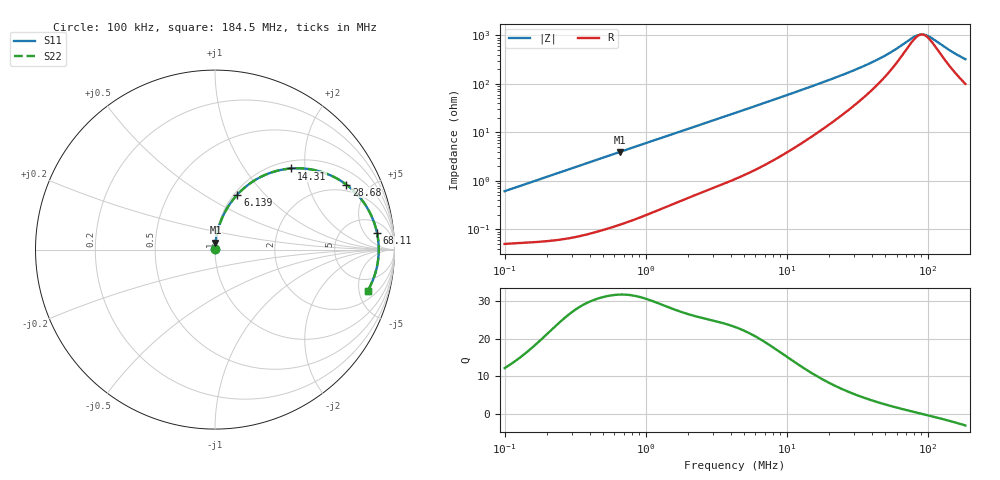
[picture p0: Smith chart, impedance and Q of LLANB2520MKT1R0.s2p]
! LLANB2520MKT1R0  S-PARAMETER MODEL  ( General Type )
! Model Generated by TAIYO YUDEN Corporation (http://www.ty-top.com)
! Version 2.0
! TAIYO YUDEN Control No. 20210629
! Copyright(c) 2012 TAIYO YUDEN CO.,LTD. All Rights Reserved.
! Product Description (link to TY-COMPAS)
! https://ds.yuden.co.jp/TYCOMPAS/or/detail?pn=LLANB2520MKT1R0M&u=M
! Products Name : Inductors
! Characteristics :
!  Inductance : 1.0 uH , SRF(min) : -Hz , DC Resistance(max) : 0.059 Ohm
!  Rated Current : Saturation :3100 mA , Temp Rise : 2700 mA (40 degC)
!  Case Size : 2.5 x 2.0 / 0.098 x 0.079 [mm/inch] , Thickness : 1.2 / 0.047 [mm/inch]
!  (Conditions: Temperature = 25 degC , DC Bias Current/Voltage = 0A / 0V)
! External Node Assignments :
!  1  o---GGG---o  2
! GND o---------o GND
! Frequency Range : 0.1MHz  -  184.468258MHz  [ 402 STEP ]
# MHz S RI R 50
! Freq[MHz].  S11 Real  S11 Imag  S21 Real  S21 Imag  S12 Real  S12 Imag  S22 Real  S22 Imag
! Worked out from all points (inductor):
!   401 points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, 100 kHz to 184.5 MHz, reference 50 ohm
!   read as one part in series: L = 966 nH near 103.8 kHz
!   highest Q = 31.7 at 655.4 kHz (marker M1), where L = 956 nH
!   self-resonance near 90.66 MHz
!   S11 on the Smith chart (normalised r, x): 100 kHz: 1.00, +0.01; 6.139 MHz: 1.03, +0.71; 14.31 MHz: 1.15, +1.68; 28.68 MHz: 1.64, +3.56; 68.11 MHz: 10, +10; 184.5 MHz: 2.99, -6.13
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0.1  0.000536 0.00607  0.9995 -0.00607  0.9995 -0.00607  0.000536 0.00607
0.352405  0.00119 0.0212  0.9988 -0.0212  0.9988 -0.0212  0.00119 0.0212
0.655361  0.00278 0.0392  0.9972 -0.0392  0.9972 -0.0392  0.00278 0.0392
1.241892  0.00791 0.0732  0.9921 -0.0732  0.9921 -0.0732  0.00791 0.0732
2.398015  0.0246 0.1367  0.9754 -0.1367  0.9754 -0.1367  0.0246 0.1367
4.294977  0.0678 0.2307  0.9322 -0.2307  0.9322 -0.2307  0.0678 0.2307
6.138922  0.1248 0.3069  0.8752 -0.3069  0.8752 -0.3069  0.1248 0.3069
9.283629  0.2403 0.3973  0.7597 -0.3973  0.7597 -0.3973  0.2403 0.3973
14.30567  0.4228 0.4519  0.5772 -0.4519  0.5772 -0.4519  0.4228 0.4519
15.13571  0.4497 0.4532  0.5503 -0.4532  0.5503 -0.4532  0.4497 0.4532
20.44747  0.5926 0.4332  0.4074 -0.4332  0.4074 -0.4332  0.5926 0.4332
28.68178  0.7316 0.3622  0.2684 -0.3622  0.2684 -0.3622  0.7316 0.3622
40.23208  0.8293 0.2615  0.1707 -0.2615  0.1707 -0.2615  0.8293 0.2615
53.33896  0.8792 0.1703  0.1208 -0.1703  0.1208 -0.1703  0.8792 0.1703
68.10626  0.9031 0.0913  0.0969 -0.0913  0.0969 -0.0913  0.9031 0.0913
77.68562  0.9097 0.0492  0.0903 -0.0492  0.0903 -0.0492  0.9097 0.0492
83.7529  0.9117 0.0252  0.0883 -0.0252  0.0883 -0.0252  0.9117 0.0252
90.29404  0.9125 0.00127  0.0875 -0.00127  0.0875 -0.00127  0.9125 0.00127
95.53302  0.9122 -0.0167  0.0878 0.0167  0.0878 0.0167  0.9122 -0.0167
106.9405  0.9095 -0.0526  0.0905 0.0526  0.0905 0.0526  0.9095 -0.0526
150.0061  0.8829 -0.1617  0.1171 0.1617  0.1171 0.1617  0.8829 -0.1617
184.4683  0.8509 -0.229  0.1491 0.229  0.1491 0.229  0.8509 -0.229
